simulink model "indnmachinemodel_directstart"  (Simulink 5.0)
settings: Solver=ode3  StartTime=0  StopTime=1.2  FixedStep=1e-5  MaxStep=10e-6  RelTol=1e-3  AbsTol=1e-6
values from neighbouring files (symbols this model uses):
  J = 0.0226    [PARAM.M]
  p = 4    [PARAM.M]
  Rr = .39    (= 0.39)    [PARAM.M]
  Rs = .19    (= 0.19)    [PARAM.M]
  wb = 2*pi*fb    (= 628.318530718)    [PARAM.M]
  Xlr = wb*Llr    (= 0.376991118431)    [PARAM.M]
  Xls = wb*Lls    (= 0.131946891451)    [PARAM.M]
  Xmstar = 1/(1/Xls+1/Xm+1/Xlr)    (= 0.0940797800005)    [PARAM.M]

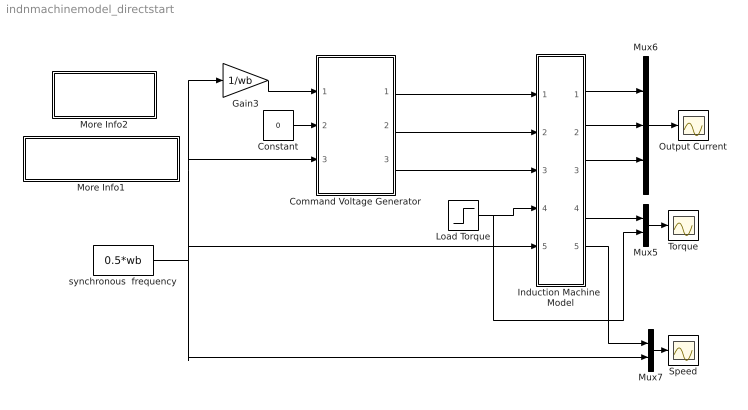
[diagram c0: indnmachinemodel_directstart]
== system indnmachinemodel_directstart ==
  Command Voltage Generator : Subsystem
  Constant : Constant  Value=0
  Gain3 : Gain  Gain=1/wb
  Induction Machine  Model : Subsystem
  Load Torque : Step  Time=.5  After=30  SampleTime=0
  More Info1 : Subsystem
  More Info2 : Subsystem
  Mux5 : Mux  Inputs=2
  Mux6 : Mux  Inputs=3
  Mux7 : Mux  Inputs=2
  Output Current : Scope
  Speed : Scope
  Torque : Scope
  synchronous  frequency : Constant  Value=0.5*wb
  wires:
  Induction Machine  Model/1(ia) -> Mux6/1
  Induction Machine  Model/2(ib) -> Mux6/2
  Induction Machine  Model/3(ic) -> Mux6/3
  Load Torque/1 -> Induction Machine  Model/4(Tl), Mux5/2
  Mux7/1 -> Speed/1
  Mux5/1 -> Torque/1
  Mux6/1 -> Output Current/1
  Constant/1 -> Command Voltage Generator/2(vds*)
  Gain3/1 -> Command Voltage Generator/1(vqs*)
  Induction Machine  Model/4(Te) -> Mux5/1
  synchronous  frequency/1 -> Gain3/1, Command Voltage Generator/3(we), Induction Machine  Model/5(we), Mux7/2
  Induction Machine  Model/5(wr) -> Mux7/1
  Command Voltage Generator/1(vao*) -> Induction Machine  Model/1(vao)
  Command Voltage Generator/2(vbo*) -> Induction Machine  Model/2(vbo)
  Command Voltage Generator/3(vco*) -> Induction Machine  Model/3(vco)

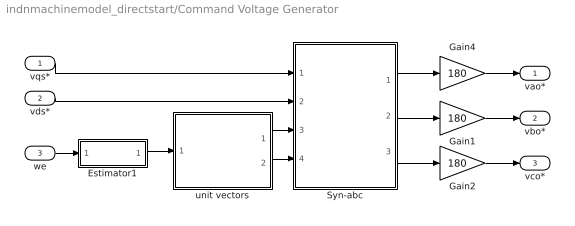
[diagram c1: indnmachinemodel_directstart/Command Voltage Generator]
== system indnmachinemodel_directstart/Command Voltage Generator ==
  vqs* : Inport
  vds* : Inport  Port=2
  we : Inport  Port=3
  Estimator1 : Subsystem
  Gain1 : Gain  Gain=180
  Gain2 : Gain  Gain=180
  Gain4 : Gain  Gain=180
  Syn-abc : Subsystem
  unit vectors : Subsystem
  vao* : Outport
  vbo* : Outport  Port=2
  vco* : Outport  Port=3
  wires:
  Syn-abc/1(vao*) -> Gain4/1
  unit vectors/1(cos(theta-e)) -> Syn-abc/3(cos(theta-e))
  unit vectors/2(sin(theta-e)) -> Syn-abc/4(sin(theta-e))
  Estimator1/1(theta-e) -> unit vectors/1(theta-e)
  we/1 -> Estimator1/1(we)
  vds*/1 -> Syn-abc/2(vds)
  vqs*/1 -> Syn-abc/1(vqs)
  Syn-abc/2(vbo*) -> Gain1/1
  Syn-abc/3(vco*) -> Gain2/1
  Gain4/1 -> vao*/1
  Gain1/1 -> vbo*/1
  Gain2/1 -> vco*/1

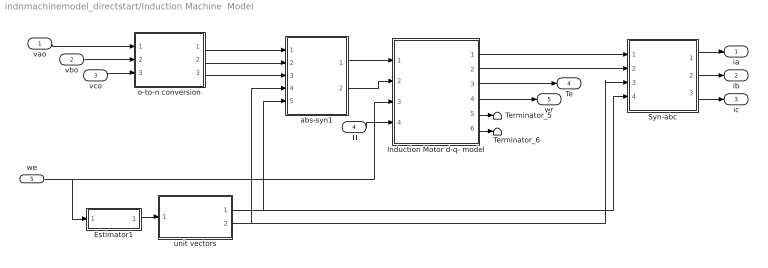
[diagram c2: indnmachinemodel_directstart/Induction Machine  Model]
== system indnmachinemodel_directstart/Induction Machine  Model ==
  vao : Inport
  vbo : Inport  Port=2
  vco : Inport  Port=3
  Tl : Inport  Port=4
  we : Inport  Port=5
  Estimator1 : Subsystem
  Induction Motor d-q- model : Subsystem
  Syn-abc : Subsystem
  Terminator_5 : Terminator
  Terminator_6 : Terminator
  abs-syn1 : Subsystem
  o-to-n conversion : Subsystem
  unit vectors : Subsystem
  ia : Outport
  ib : Outport  Port=2
  ic : Outport  Port=3
  Te : Outport  Port=4
  wr : Outport  Port=5
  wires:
  we/1 -> Induction Motor d-q- model/3(we), Estimator1/1(we)
  Estimator1/1(theta-e) -> unit vectors/1(theta-e)
  Induction Motor d-q- model/6("iqr ") -> Terminator_6/1
  Tl/1 -> Induction Motor d-q- model/4(Tl)
  Syn-abc/2(ib) -> ib/1
  Syn-abc/3(ic) -> ic/1
  Induction Motor d-q- model/5("idr ") -> Terminator_5/1
  Syn-abc/1(ia) -> ia/1
  Induction Motor d-q- model/3("Te ") -> Te/1
  Induction Motor d-q- model/4("wr ") -> wr/1
  vao/1 -> o-to-n conversion/1(vao)
  vbo/1 -> o-to-n conversion/2(vbo)
  vco/1 -> o-to-n conversion/3(vco)
  unit vectors/1(sin(theta-e)) -> Syn-abc/4(sin(theta-e)), abs-syn1/5(sin(theta-e))
  unit vectors/2(cos(theta-e)) -> Syn-abc/3(cos(theta-e)), abs-syn1/4(cos(theta-e))
  Induction Motor d-q- model/2("ids ") -> Syn-abc/2(ids)
  Induction Motor d-q- model/1("iqs ") -> Syn-abc/1(iqs)
  o-to-n conversion/1(van) -> abs-syn1/1(van)
  o-to-n conversion/2(vbn) -> abs-syn1/2(vbn)
  o-to-n conversion/3(vcn) -> abs-syn1/3(vcn)
  abs-syn1/2(vds) -> Induction Motor d-q- model/2(vds)
  abs-syn1/1(vqs) -> Induction Motor d-q- model/1(vqs)

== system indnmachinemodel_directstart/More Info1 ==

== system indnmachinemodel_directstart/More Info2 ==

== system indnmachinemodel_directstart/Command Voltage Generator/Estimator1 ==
  we : Inport
  Constant : Constant  Value=2*pi
  Integrator : Integrator
  Math Function3 : Math  Operator=mod
  theta-e : Outport
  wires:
  Math Function3/1 -> theta-e/1
  Integrator/1 -> Math Function3/1
  Constant/1 -> Math Function3/2
  we/1 -> Integrator/1

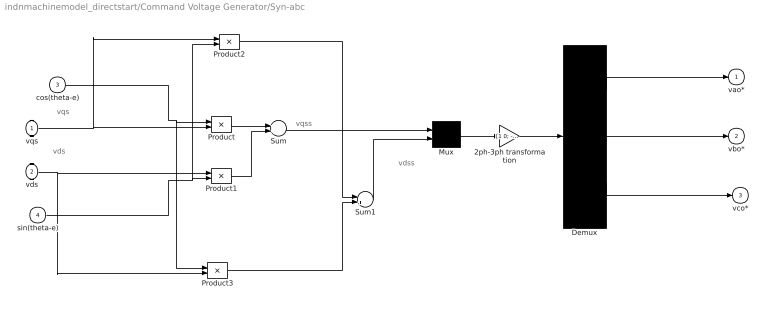
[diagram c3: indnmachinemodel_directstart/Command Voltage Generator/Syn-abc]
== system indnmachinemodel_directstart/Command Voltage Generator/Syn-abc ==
  note: vqss
  note: vqs
  note: vdss
  note: vds
  vqs : Inport
  vds : Inport  Port=2
  cos(theta-e) : Inport  Port=3
  sin(theta-e) : Inport  Port=4
  2ph-3ph transformation : Gain  Gain="[1 0; -1/2 -sqrt(3)/2;  -1/2 sqrt(3)/2]"  Multiplication=Matrix(K*u)
  Demux : Demux  Outputs=3
  Mux : Mux  Inputs=2
  Product{,1..3} (4 alike) : Product
  Sum : Sum
  Sum1 : Sum  Inputs=-+
  vao* : Outport
  vbo* : Outport  Port=2
  vco* : Outport  Port=3
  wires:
  2ph-3ph transformation/1 -> Demux/1
  Sum1/1 -> Mux/2
  Product/1 -> Sum/1
  Product1/1 -> Sum/2
  sin(theta-e)/1 -> Product2/2, Product1/2
  cos(theta-e)/1 -> Product3/1, Product/1
  Product3/1 -> Sum1/2
  Product2/1 -> Sum1/1
  Mux/1 -> 2ph-3ph transformation/1
  vds/1 -> Product3/2, Product1/1
  vqs/1 -> Product2/1, Product/2
  Demux/1 -> vao*/1
  Demux/2 -> vbo*/1
  Demux/3 -> vco*/1
  Sum/1 -> Mux/1

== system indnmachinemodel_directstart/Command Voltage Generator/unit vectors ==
  theta-e : Inport
  Trigonometric Function : Trigonometry
  Trigonometric Function1 : Trigonometry  Operator=cos
  cos(theta-e) : Outport
  sin(theta-e) : Outport  Port=2
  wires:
  Trigonometric Function/1 -> sin(theta-e)/1
  Trigonometric Function1/1 -> cos(theta-e)/1
  theta-e/1 -> Trigonometric Function1/1, Trigonometric Function/1

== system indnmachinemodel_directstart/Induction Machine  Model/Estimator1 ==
  we : Inport
  Constant : Constant  Value=2*pi
  Integrator : Integrator  InitialCondition=0.01
  Math Function3 : Math  Operator=mod
  theta-e : Outport
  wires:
  we/1 -> Integrator/1
  Constant/1 -> Math Function3/2
  Integrator/1 -> Math Function3/1
  Math Function3/1 -> theta-e/1

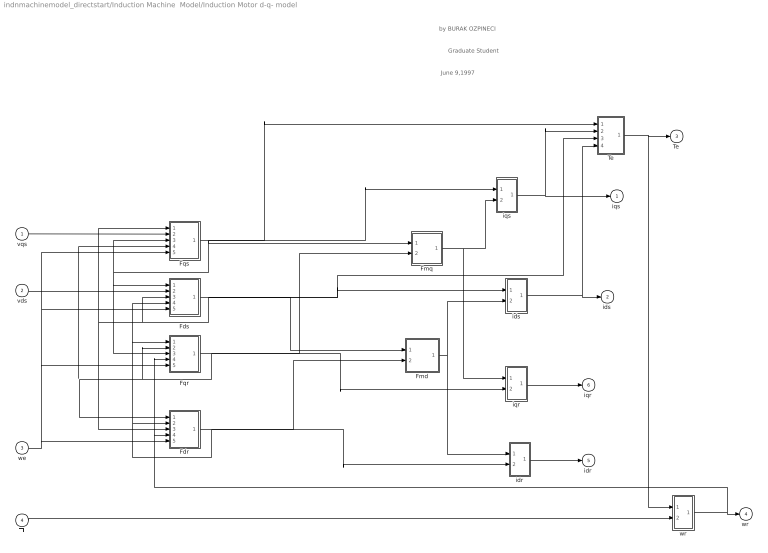
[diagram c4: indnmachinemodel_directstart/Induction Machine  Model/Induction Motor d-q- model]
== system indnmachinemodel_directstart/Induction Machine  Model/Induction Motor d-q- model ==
  note: by BURAK OZPINECI
  note: Graduate Student
  note: June 9,1997
  vqs : Inport
  vds : Inport  Port=2
  we : Inport  Port=3
  Tl : Inport  Port=4
  Fdr : Subsystem
  Fds : Subsystem
  Fmd : Subsystem
  Fmq : Subsystem
  Fqr : Subsystem
  Fqs : Subsystem
  Te : Subsystem
  idr : Subsystem
  ids : Subsystem
  iqr : Subsystem
  iqs : Subsystem
  wr : Subsystem
  "iqs " : Outport
  "ids " : Outport  Port=2
  "Te " : Outport  Port=3
  "wr " : Outport  Port=4
  "idr " : Outport  Port=5
  "iqr " : Outport  Port=6
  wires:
  Fdr/1("Fdr ") -> idr/2(Fdr), Fdr/2(Fdr), Fqr/1(Fdr), Fds/4(Fdr), Fmd/2(Fdr)
  we/1 -> Fqs/5(we), Fds/5(we), Fqr/5(we), Fdr/5(we)
  wr/1(wr) -> "wr "/1, Fqr/4(wr), Fdr/4(wr)
  vqs/1 -> Fqs/2(Vqs)
  vds/1 -> Fds/2(Vds)
  Tl/1 -> wr/2(Tl)
  Fqs/1("Fqs ") -> Fqs/3(Fqs), Fqr/3(Fqs), Fds/1(Fqs), Fmq/1(Fqs), iqs/1(Fqs), Te/1(Fqs)
  Fqr/1("Fqr ") -> Fqr/2(Fqr), Fqs/4(Fqr), Fdr/1(Fqr), iqr/2(Fqr), Fmq/2(Fqr)
  Fds/1("Fds ") -> Fds/3(Fds), Fqs/1(Fds), Fdr/3(Fds), Fmd/1(Fds), ids/1(Fds), Te/3(Fds)
  iqr/1(iqr) -> "iqr "/1
  Fmq/1(Fmq) -> iqs/2(Fmq), iqr/1(Fmq)
  idr/1(idr) -> "idr "/1
  Fmd/1(Fmd) -> ids/2(Fmd), idr/1(Fmd)
  Te/1(Te) -> "Te "/1, wr/1(Te)
  ids/1(ids) -> "ids "/1, Te/4(ids)
  iqs/1(iqs) -> "iqs "/1, Te/2(iqs)

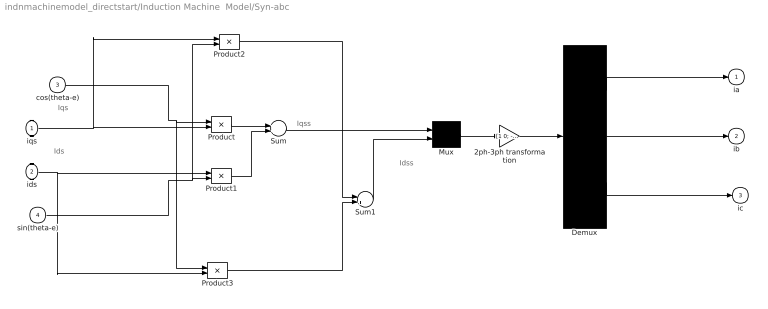
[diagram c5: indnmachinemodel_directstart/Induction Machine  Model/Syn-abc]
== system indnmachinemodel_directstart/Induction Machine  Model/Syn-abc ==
  note: Iqss
  note: Iqs
  note: Idss
  note: Ids
  iqs : Inport
  ids : Inport  Port=2
  cos(theta-e) : Inport  Port=3
  sin(theta-e) : Inport  Port=4
  2ph-3ph transformation : Gain  Gain="[1 0; -1/2 -sqrt(3)/2;  -1/2 sqrt(3)/2]"  Multiplication=Matrix(K*u)
  Demux : Demux  Outputs=3
  Mux : Mux  Inputs=2
  Product{,1..3} (4 alike) : Product
  Sum : Sum
  Sum1 : Sum  Inputs=-+
  ia : Outport
  ib : Outport  Port=2
  ic : Outport  Port=3
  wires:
  2ph-3ph transformation/1 -> Demux/1
  Sum1/1 -> Mux/2
  Sum/1 -> Mux/1
  Product/1 -> Sum/1
  Product1/1 -> Sum/2
  sin(theta-e)/1 -> Product2/2, Product1/2
  cos(theta-e)/1 -> Product3/1, Product/1
  Product3/1 -> Sum1/2
  Product2/1 -> Sum1/1
  Mux/1 -> 2ph-3ph transformation/1
  ids/1 -> Product3/2, Product1/1
  iqs/1 -> Product2/1, Product/2
  Demux/1 -> ia/1
  Demux/2 -> ib/1
  Demux/3 -> ic/1

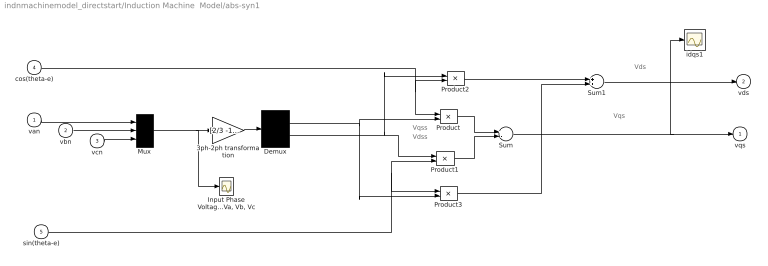
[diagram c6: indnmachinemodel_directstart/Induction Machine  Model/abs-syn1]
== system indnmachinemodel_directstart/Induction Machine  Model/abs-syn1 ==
  note: Vqs
  note: Vds
  note: Vqss
  note: Vdss
  van : Inport
  vbn : Inport  Port=2
  vcn : Inport  Port=3
  cos(theta-e) : Inport  Port=4
  sin(theta-e) : Inport  Port=5
  3ph-2ph transformation : Gain  Gain=[2/3 -1/3 -1/3;0 -1/sqrt(3) 1/sqrt(3)]  Multiplication=Matrix(K*u)
  Demux : Demux  Outputs=2
  "Input Phase Voltages Va, Vb, Vc" : Scope
  Mux : Mux  Inputs=3
  Product{,1..3} (4 alike) : Product
  Sum : Sum  Inputs=+-
  Sum1 : Sum
  idqs1 : Scope
  vqs : Outport
  vds : Outport  Port=2
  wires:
  cos(theta-e)/1 -> Product2/2, Product/1
  sin(theta-e)/1 -> Product3/1, Product1/2
  Demux/1 -> Product3/2, Product/2
  van/1 -> Mux/1
  Demux/2 -> Product1/1, Product2/1
  vbn/1 -> Mux/2
  Product3/1 -> Sum1/2
  Product2/1 -> Sum1/1
  Sum/1 -> idqs1/1, vqs/1
  Sum1/1 -> vds/1
  Product1/1 -> Sum/2
  Mux/1 -> 3ph-2ph transformation/1, "Input Phase Voltages Va, Vb, Vc"/1
  vcn/1 -> Mux/3
  Product/1 -> Sum/1
  3ph-2ph transformation/1 -> Demux/1

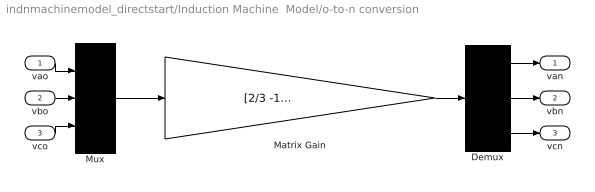
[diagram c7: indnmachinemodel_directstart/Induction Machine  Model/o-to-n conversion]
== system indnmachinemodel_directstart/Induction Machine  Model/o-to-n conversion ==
  vao : Inport
  vbo : Inport  Port=2
  vco : Inport  Port=3
  Demux : Demux  Outputs=3
  Matrix Gain : Gain  Gain=[2/3 -1/3 -1/3; -1/3 2/3 -1/3; -1/3 -1/3 2/3]  Multiplication=Matrix(K*u)
  Mux : Mux  Inputs=3
  van : Outport
  vbn : Outport  Port=2
  vcn : Outport  Port=3
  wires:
  Demux/3 -> vcn/1
  Demux/2 -> vbn/1
  Demux/1 -> van/1
  vco/1 -> Mux/3
  vbo/1 -> Mux/2
  vao/1 -> Mux/1
  Matrix Gain/1 -> Demux/1
  Mux/1 -> Matrix Gain/1

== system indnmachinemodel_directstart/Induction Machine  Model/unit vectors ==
  theta-e : Inport
  Trigonometric Function : Trigonometry
  Trigonometric Function1 : Trigonometry  Operator=cos
  sin(theta-e) : Outport
  cos(theta-e) : Outport  Port=2
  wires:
  theta-e/1 -> Trigonometric Function/1, Trigonometric Function1/1
  Trigonometric Function1/1 -> cos(theta-e)/1
  Trigonometric Function/1 -> sin(theta-e)/1

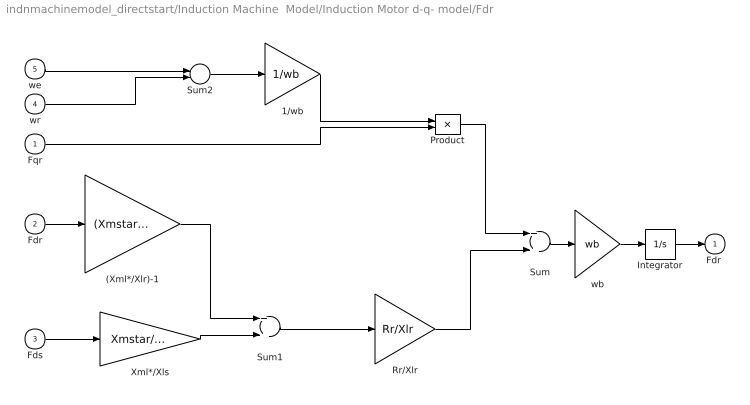
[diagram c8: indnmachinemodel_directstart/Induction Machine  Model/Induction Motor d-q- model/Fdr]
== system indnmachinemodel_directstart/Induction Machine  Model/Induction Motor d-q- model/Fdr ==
  Fqr : Inport
  Fdr : Inport  Port=2
  Fds : Inport  Port=3
  wr : Inport  Port=4
  we : Inport  Port=5
  (Xml*/Xlr)-1 : Gain  Gain=(Xmstar/Xlr)-1
  1/wb : Gain  Gain=1/wb
  Integrator : Integrator
  Product : Product
  Rr/Xlr : Gain  Gain=Rr/Xlr
  Sum : Sum
  Sum1 : Sum
  Sum2 : Sum  Inputs=+-
  Xml*/Xls : Gain  Gain=Xmstar/Xls
  wb : Gain  Gain=wb
  "Fdr " : Outport
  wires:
  Rr/Xlr/1 -> Sum/2
  Xml*/Xls/1 -> Sum1/2
  (Xml*/Xlr)-1/1 -> Sum1/1
  Product/1 -> Sum/1
  1/wb/1 -> Product/1
  wr/1 -> Sum2/2
  Fqr/1 -> Product/2
  we/1 -> Sum2/1
  Sum2/1 -> 1/wb/1
  Fds/1 -> Xml*/Xls/1
  Integrator/1 -> "Fdr "/1
  Fdr/1 -> (Xml*/Xlr)-1/1
  Sum1/1 -> Rr/Xlr/1
  Sum/1 -> wb/1
  wb/1 -> Integrator/1

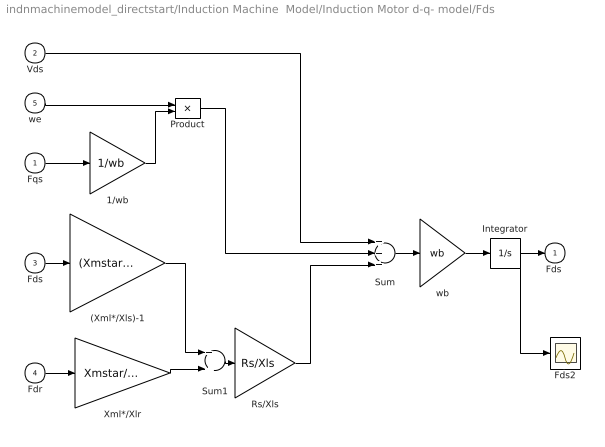
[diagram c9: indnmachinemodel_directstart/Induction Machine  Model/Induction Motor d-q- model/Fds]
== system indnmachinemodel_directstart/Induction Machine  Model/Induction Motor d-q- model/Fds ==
  Fqs : Inport
  Vds : Inport  Port=2
  Fds : Inport  Port=3
  Fdr : Inport  Port=4
  we : Inport  Port=5
  (Xml*/Xls)-1 : Gain  Gain=(Xmstar/Xls)-1
  1/wb : Gain  Gain=1/wb
  Fds2 : Scope
  Integrator : Integrator
  Product : Product
  Rs/Xls : Gain  Gain=Rs/Xls
  Sum : Sum  Inputs=+++
  Sum1 : Sum
  Xml*/Xlr : Gain  Gain=Xmstar/Xlr
  wb : Gain  Gain=wb
  "Fds " : Outport
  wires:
  1/wb/1 -> Product/2
  Product/1 -> Sum/2
  we/1 -> Product/1
  wb/1 -> Integrator/1
  Fdr/1 -> Xml*/Xlr/1
  Fds/1 -> (Xml*/Xls)-1/1
  Vds/1 -> Sum/1
  Fqs/1 -> 1/wb/1
  Rs/Xls/1 -> Sum/3
  (Xml*/Xls)-1/1 -> Sum1/1
  Xml*/Xlr/1 -> Sum1/2
  Sum1/1 -> Rs/Xls/1
  Sum/1 -> wb/1
  Integrator/1 -> "Fds "/1, Fds2/1

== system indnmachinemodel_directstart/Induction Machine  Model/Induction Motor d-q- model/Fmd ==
  Fds : Inport
  Fdr : Inport  Port=2
  Sum8 : Sum
  Xmstar/Xlr : Gain  Gain=Xmstar/Xlr
  Xmstar/Xls : Gain  Gain=Xmstar/Xls
  Fmd : Outport
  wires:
  Fdr/1 -> Xmstar/Xlr/1
  Sum8/1 -> Fmd/1
  Fds/1 -> Xmstar/Xls/1
  Xmstar/Xls/1 -> Sum8/1
  Xmstar/Xlr/1 -> Sum8/2

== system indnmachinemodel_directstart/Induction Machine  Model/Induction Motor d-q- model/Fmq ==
  Fqs : Inport
  Fqr : Inport  Port=2
  Sum8 : Sum
  Xmstar/Xlr : Gain  Gain=Xmstar/Xlr
  Xmstar/Xls : Gain  Gain=Xmstar/Xls
  Fmq : Outport
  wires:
  Fqr/1 -> Xmstar/Xlr/1
  Sum8/1 -> Fmq/1
  Fqs/1 -> Xmstar/Xls/1
  Xmstar/Xls/1 -> Sum8/1
  Xmstar/Xlr/1 -> Sum8/2

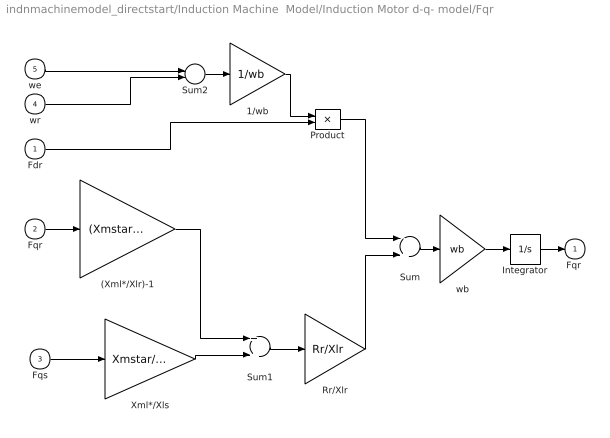
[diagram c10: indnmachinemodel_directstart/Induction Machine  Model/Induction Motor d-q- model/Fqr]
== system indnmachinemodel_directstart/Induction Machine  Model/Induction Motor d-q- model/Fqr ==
  Fdr : Inport
  Fqr : Inport  Port=2
  Fqs : Inport  Port=3
  wr : Inport  Port=4
  we : Inport  Port=5
  (Xml*/Xlr)-1 : Gain  Gain=(Xmstar/Xlr)-1
  1/wb : Gain  Gain=1/wb
  Integrator : Integrator
  Product : Product
  Rr/Xlr : Gain  Gain=Rr/Xlr
  Sum : Sum  Inputs=-+
  Sum1 : Sum
  Sum2 : Sum  Inputs=+-
  Xml*/Xls : Gain  Gain=Xmstar/Xls
  wb : Gain  Gain=wb
  "Fqr " : Outport
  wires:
  (Xml*/Xlr)-1/1 -> Sum1/1
  Rr/Xlr/1 -> Sum/2
  Product/1 -> Sum/1
  Fdr/1 -> Product/2
  1/wb/1 -> Product/1
  Sum2/1 -> 1/wb/1
  wr/1 -> Sum2/2
  we/1 -> Sum2/1
  Fqs/1 -> Xml*/Xls/1
  Integrator/1 -> "Fqr "/1
  Fqr/1 -> (Xml*/Xlr)-1/1
  Xml*/Xls/1 -> Sum1/2
  Sum1/1 -> Rr/Xlr/1
  Sum/1 -> wb/1
  wb/1 -> Integrator/1

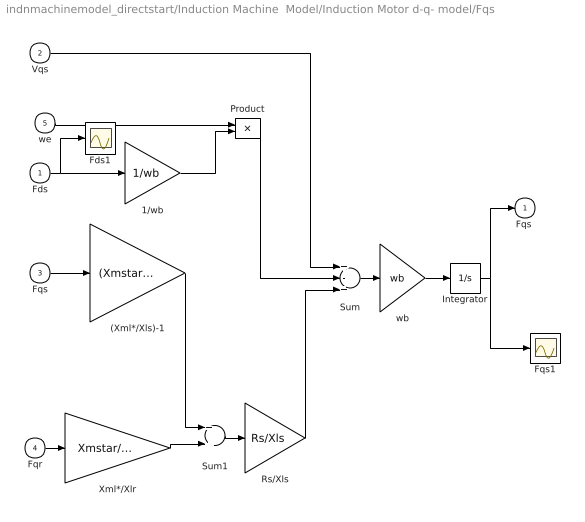
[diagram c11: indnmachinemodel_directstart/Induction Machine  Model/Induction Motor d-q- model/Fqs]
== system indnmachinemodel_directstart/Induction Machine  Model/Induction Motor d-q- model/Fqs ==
  Fds : Inport
  Vqs : Inport  Port=2
  Fqs : Inport  Port=3
  Fqr : Inport  Port=4
  we : Inport  Port=5
  (Xml*/Xls)-1 : Gain  Gain=(Xmstar/Xls)-1
  1/wb : Gain  Gain=1/wb
  Fds1 : Scope
  Fqs1 : Scope
  Integrator : Integrator
  Product : Product
  Rs/Xls : Gain  Gain=Rs/Xls
  Sum : Sum  Inputs=+-+
  Sum1 : Sum
  Xml*/Xlr : Gain  Gain=Xmstar/Xlr
  wb : Gain  Gain=wb
  "Fqs " : Outport
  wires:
  1/wb/1 -> Product/2
  Product/1 -> Sum/2
  we/1 -> Product/1
  Xml*/Xlr/1 -> Sum1/2
  (Xml*/Xls)-1/1 -> Sum1/1
  wb/1 -> Integrator/1
  Fqr/1 -> Xml*/Xlr/1
  Fqs/1 -> (Xml*/Xls)-1/1
  Vqs/1 -> Sum/1
  Rs/Xls/1 -> Sum/3
  Sum1/1 -> Rs/Xls/1
  Sum/1 -> wb/1
  Integrator/1 -> "Fqs "/1, Fqs1/1
  Fds/1 -> 1/wb/1, Fds1/1

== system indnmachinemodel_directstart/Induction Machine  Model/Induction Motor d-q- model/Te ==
  Fqs : Inport
  iqs : Inport  Port=2
  Fds : Inport  Port=3
  ids : Inport  Port=4
  3*p/(4*wb) : Gain  Gain=3*p/(4*wb)
  Product : Product
  Product1 : Product
  Sum7 : Sum  Inputs=+-
  Te : Outport
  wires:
  ids/1 -> Product/2
  Fqs/1 -> Product/1
  iqs/1 -> Product1/2
  Fds/1 -> Product1/1
  3*p/(4*wb)/1 -> Te/1
  Sum7/1 -> 3*p/(4*wb)/1
  Product1/1 -> Sum7/1
  Product/1 -> Sum7/2

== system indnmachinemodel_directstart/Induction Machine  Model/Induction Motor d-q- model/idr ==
  Fmd : Inport
  Fdr : Inport  Port=2
  1/Xlr : Gain  Gain=1/Xlr
  Sum8 : Sum  Inputs=+-
  idr : Outport
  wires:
  Fmd/1 -> Sum8/2
  1/Xlr/1 -> idr/1
  Fdr/1 -> Sum8/1
  Sum8/1 -> 1/Xlr/1

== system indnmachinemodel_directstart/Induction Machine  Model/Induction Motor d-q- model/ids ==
  Fds : Inport
  Fmd : Inport  Port=2
  1/Xls : Gain  Gain=1/Xls
  Sum8 : Sum  Inputs=+-
  ids : Outport
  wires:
  Fmd/1 -> Sum8/2
  1/Xls/1 -> ids/1
  Fds/1 -> Sum8/1
  Sum8/1 -> 1/Xls/1

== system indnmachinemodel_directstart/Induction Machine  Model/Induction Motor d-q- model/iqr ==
  Fmq : Inport
  Fqr : Inport  Port=2
  1/Xlr : Gain  Gain=1/Xlr
  Sum8 : Sum  Inputs=+-
  iqr : Outport
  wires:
  Fmq/1 -> Sum8/2
  1/Xlr/1 -> iqr/1
  Fqr/1 -> Sum8/1
  Sum8/1 -> 1/Xlr/1

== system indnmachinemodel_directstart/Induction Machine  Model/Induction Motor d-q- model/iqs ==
  Fqs : Inport
  Fmq : Inport  Port=2
  1/Xls : Gain  Gain=1/Xls
  Sum8 : Sum  Inputs=+-
  iqs : Outport
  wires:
  Fmq/1 -> Sum8/2
  1/Xls/1 -> iqs/1
  Fqs/1 -> Sum8/1
  Sum8/1 -> 1/Xls/1

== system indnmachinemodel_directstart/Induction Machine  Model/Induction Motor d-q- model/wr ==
  Te : Inport
  Tl : Inport  Port=2
  Integrator : Integrator
  Sum7 : Sum  Inputs=+-
  p/(2*J) : Gain  Gain=p/(2*J)
  wr : Outport
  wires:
  Te/1 -> Sum7/1
  Tl/1 -> Sum7/2
  Integrator/1 -> wr/1
  p/(2*J)/1 -> Integrator/1
  Sum7/1 -> p/(2*J)/1
